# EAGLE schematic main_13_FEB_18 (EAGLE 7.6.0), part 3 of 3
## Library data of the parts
IC1 IC4-IC7 IC16 IC17 IC21 IC48 IC82 IC86 IC88 IC93 IC98-IC101 IC118 IC123 IC153 IC165 IC166 IC169 IC173 IC180 IC184 IC185 IC189 IC202 IC205 IC216 IC217 IC233 IC234 IC239 IC240 IC246 IC251 IC254 IC261 IC262 IC265 IC296 IC301 = 74xx-us:74*377: Octal D type FLIP FLOP, enable
IC2 IC3 IC9 IC19 IC28 IC102-IC104 IC113-IC117 IC122 IC125 IC140 IC145 IC146 IC154 IC171 IC210 IC215 IC245 IC252 IC253 IC259 IC260 IC263 IC264 IC266 IC267 IC302 IC303 = 74xx-us:74*541: Octal BUFFER and LINE DRIVER, 3-state; OC_FARNELL: unknown
IC8 IC163 IC164 IC168 IC174 IC187 IC188 IC204 IC221 = 74xx-us:74*74: Dual D type positive edge triggered FLIP FLOP, preset and clear
IC10-IC13 IC24-IC27 IC30 IC31 IC69 IC105-IC112 IC176 IC178 IC179 IC181-IC183 IC244 IC247 IC288-IC295 IC297-IC300 = 74xx-us:74*244: Octal BUFFER and LINE DRIVER, 3-state; MF: TEXAS INSTRUMENTS; MPN: SN74LS244N; OC_FARNELL: 1739688
IC14 IC15 = 74xx-us:74*181: ARITHMETIC LOGIC UNIT function generator; OC_FARNELL: unknown
IC18 IC46 IC67 IC81 IC147 IC170 IC250 = 74xx-us:74*32: Quad 2-input OR gate; MF: TEXAS INSTRUMENTS; MPN: SN7432N; OC_FARNELL: 1607803
IC20 IC34-IC38 IC40 IC41 IC70 IC71 IC73 IC129 IC142 IC159 IC160 IC172 IC186 = 74xx-us:74*151: Data SELECTOR/MULTIPLEXER
IC22 IC23 IC94-IC97 IC121 IC167 IC257 IC258 = 74xx-us:74*157: Quadruple 2-line to 1-line data SELECTOR/MULTIPLEXER; OC_FARNELL: unknown
IC32 IC33 IC60-IC62 IC75-IC79 IC134-IC137 = 74xx-us:74*273: Octal D type FLIP FLOP, clear; OC_FARNELL: unknown
IC39 IC42 IC45 IC47 IC120 IC124 IC127 IC133 IC143 IC148 IC161 IC195 IC207 IC218-IC220 IC223-IC225 IC269 = 74xx-us:74*08: Quad 2-input AND gate; OC_FARNELL: unknown
IC43 IC54 IC57 IC59 IC83 IC84 IC119 IC198 = 74xx-us:74*04: Hex INVERTER; OC_FARNELL: unknown
IC44 = 74xx-us:74*74: Dual D type positive edge triggered FLIP FLOP, preset and clear; OC_FARNELL: unknown
IC49 IC55 IC63 IC68 = 74xx-us:74*257: Quadruple 2-to 1 line data SELECTOR/MULTIPLEXER; OC_FARNELL: unknown
IC50-IC53 IC283-IC287 = 74xx-us:74*283: 4-bit binary FULL ADDER, fast carry; OC_FARNELL: unknown
IC56 IC155 IC156 IC208 IC241 IC243 IC255 IC256 = 74xx-us:74*153: Dual 4-line to 1-line data SELECTOR/MULTIPLEXER; OC_FARNELL: unknown
IC58 IC72 IC74 IC80 IC130 IC175 IC177 IC192-IC194 IC200 IC209 = 74xx-us:74*86: Quad 2-input EXCLUSIV-OR (XOR) gate; OC_FARNELL: unknown
IC64 IC85 IC132 IC138 IC150 IC151 IC157 IC158 IC191 = 74xx-us:74*10: Triple 3-input NAND gate
IC65 IC66 IC131 = 74xx-us:74*02: Quad 2-input NOR gate
IC87 = 74xx-us:74*279: Quadruple S-R LATCH; OC_FARNELL: unknown
IC89-IC92 IC211-IC214 IC229-IC232 IC235-IC238 = 74xx-us:74*244: Octal BUFFER and LINE DRIVER, 3-state; OC_FARNELL: unknown
IC126 = 74xx-us:74*377: Octal D type FLIP FLOP, enable; OC_FARNELL: unknown
IC128 IC144 IC248 IC249 = 74xx-us:74*173: 4-bit D type REGISTER, 3-state
IC139 = 74xx-us:74*173: 4-bit D type REGISTER, 3-state; OC_FARNELL: unknown
IC141 = 74xx-us:74*11: Triple 3-input AND gate
IC149 IC196 IC270 IC271 = 74xx-us:74*04: Hex INVERTER
IC152 IC190 IC201 IC203 IC206 IC228 IC242 = 74xx-us:74*00: Quad 2-input NAND gate
IC162 IC227 = 74xx-us:74*273: Octal D type FLIP FLOP, clear
IC197 IC199 = 74xx-us:74*260: Dual 5-input positive NOR gate; OC_FARNELL: unknown
IC222 = 74xx-us:74*138: 3-line to 8-line DECODER/DEMULTIPLEXER
IC226 = 74xx-us:74*148: 10-line to 4-line and 8-line to 3-line PRIORITY ENCODER
IC268 IC272 IC277 IC278 = 74xx-us:74*257: Quadruple 2-to 1 line data SELECTOR/MULTIPLEXER
IC273-IC276 IC279-IC282 = 74xx-us:74*253: Dual 4-to 1 line data SELECTOR/MULTIPLEXER, 3-state
R1-R3 R9 = rcl:R-US_: RESISTOR, American symbol; OC_FARNELL: unknown
R5-R8 R10-R14 = resistor:R-US_: RESISTOR, American symbol
RN1-RN5 = resistor-dil:8R-N: DIL RESISTOR; OC_FARNELL: unknown; OC_NEWARK: unknown
S1 S2 S4 = switch:TL36PO: TINY SWITCH ON - ON Source: http://www2.produktinfo.conrad.com/datenblaetter/700000-724999/705152-da-01-de-Subminiaturschalter_TL_36YO.pdf; OC_FARNELL: unknown
SW3 = special:SW-C10: SWITCH 10-step rotary switch; OC_FARNELL: unknown
U$1-U$12 = atmel_28c:AT28C256-28DIP: IC EEPROM 256KBIT 150NS 28DIP; OC_FARNELL: unknown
